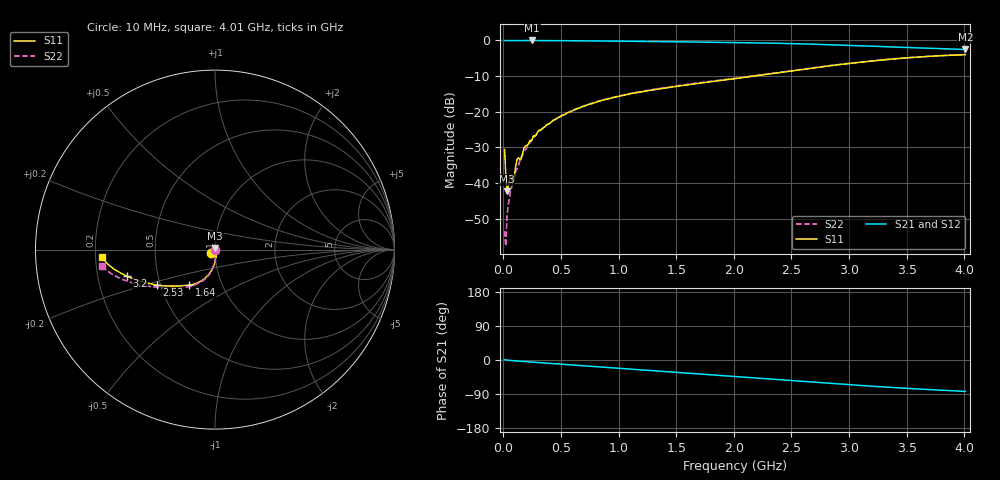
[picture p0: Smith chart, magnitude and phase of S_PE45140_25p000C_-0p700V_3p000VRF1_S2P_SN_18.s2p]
! Device ID: PE45140
! Serial: 18
! Temp: 25.00C
! VDD: 3.000
! VCTRL: -0.700
! Control_Hi: 3.000
! Control_Lo: 0.000
! Logic State: LS_RF1
! Port 1: RF1
! Port 2: RF2
! ThroughPath:1-2
! IDD: 2.08088917e-010
! ISS: 8.76524355e-011
#  Hz  S  RI  R  50
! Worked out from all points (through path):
!   401 points, 10 MHz to 4.01 GHz, reference 50 ohm
!   highest |S21| = -0.02 dB at 250 MHz (marker M1); lowest = -2.5 dB at 4.01 GHz (marker M2)
!   group delay of S21, straight-line fit = 58.9 ps
!   lowest |S11| = -42.4 dB at 30 MHz (marker M3), VSWR 1.02, Z = 50.1 + j0.754 ohm
!   |S11| at or under -10 dB: start of sweep to 2.179 GHz
!   |S22| runs from -57.7 to -4.0 dB; largest |S21 - S12| = 0.022
!   S11 on the Smith chart (normalised r, x): 10 MHz: 0.96, -0.04; 1.64 GHz: 0.70, -0.29; 2.53 GHz: 0.48, -0.22; 3.2 GHz: 0.33, -0.13; 4.01 GHz: 0.23, -0.03
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1e7  -0.0224 -0.0192  0.9934 0.01  0.9981 -0.0115  -0.000811 -0.00196
3e7  0.00131 0.00752  0.9952 -0.00421  1 -0.0156  0.00298 -0.00142
4e7  0.00854 0.000436  0.9966 -0.01  0.9987 -0.0194  0.00355 -0.00338
5e7  0.00785 -0.0079  0.997 -0.0151  0.9984 -0.0228  0.00322 -0.00496
9e7  0.00372 -0.0103  0.997 -0.0325  0.9967 -0.0367  0.00266 -0.0112
1.1e8  0.00697 -0.0173  0.9967 -0.0416  0.9961 -0.0437  0.00315 -0.0148
1.3e8  0.00424 -0.0222  0.9955 -0.0501  0.9957 -0.051  0.00291 -0.0175
1.7e8  0.00624 -0.027  0.9941 -0.0647  0.9948 -0.0665  0.00359 -0.0254
1.9e8  0.00427 -0.0327  0.9932 -0.0728  0.9936 -0.0741  0.00249 -0.0288
2.5e8  0.00677 -0.0409  0.9934 -0.0941  0.9913 -0.0987  0.00296 -0.0405
3.3e8  0.00124 -0.0561  0.985 -0.1258  0.9862 -0.1269  0.00109 -0.0567
4.4e8  -0.00392 -0.0771  0.9771 -0.1676  0.978 -0.168  -0.003 -0.0764
6.8e8  -0.0193 -0.1155  0.952 -0.255  0.9522 -0.2547  -0.0175 -0.1166
9.8e8  -0.0499 -0.1543  0.9085 -0.3562  0.9093 -0.3555  -0.0468 -0.1568
1.35e9  -0.097 -0.1849  0.8393 -0.4707  0.8401 -0.4706  -0.0954 -0.1889
1.64e9  -0.1428 -0.1971  0.7739 -0.5519  0.7748 -0.5517  -0.1388 -0.2047
2.01e9  -0.2093 -0.2031  0.6767 -0.6428  0.6777 -0.6429  -0.2033 -0.2135
2.53e9  -0.3231 -0.1971  0.5138 -0.7376  0.5153 -0.7373  -0.3195 -0.2097
2.68e9  -0.3612 -0.1894  0.4631 -0.7546  0.4647 -0.7543  -0.3563 -0.2067
3.2e9  -0.4919 -0.1473  0.2937 -0.7756  0.2961 -0.7755  -0.486 -0.1771
3.35e9  -0.5261 -0.1299  0.2496 -0.7728  0.2521 -0.7729  -0.5199 -0.1651
4.01e9  -0.6298 -0.0398  0.0914 -0.7404  0.0933 -0.7413  -0.627 -0.0931
